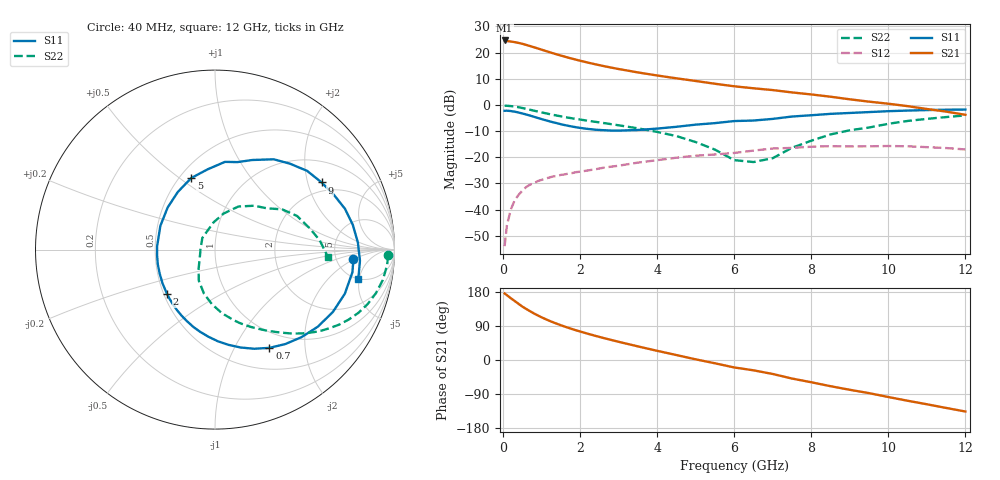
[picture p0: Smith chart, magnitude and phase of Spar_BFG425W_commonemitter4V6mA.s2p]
! Filename: 46bfg425.001
! BFG425W Field C1
! V1=8.248E-001V,V2=4.000E+000V, I1=6.283E-005A, I2=6.010E-003A
# GHz  S  MA  R 50
!  S11  S21  S12  S22
!Freq(GHz)  Mag  Ang  Mag  Ang  Mag  Ang  Mag  Ang
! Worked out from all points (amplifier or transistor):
!   44 points, 40 MHz to 12 GHz, reference 50 ohm
!   highest |S21| = 24.6 dB at 40 MHz (marker M1)
!   |S21| within 3 dB of that: start of sweep to 889.8 MHz
!   unconditionally stable (mu >= 1): 2.289 GHz to end of sweep
!   at 700 MHz: K = 0.40, MSG = 26.5 dB, |S12| = -30.5 dB
!   at 2.4 GHz: K = 1.03, MAG = 19.0 dB, |S12| = -24.6 dB
!   at 12 GHz: K = 1.47, MAG = 2.6 dB, |S12| = -17.0 dB
!   S11 on the Smith chart (normalised r, x): 40 MHz: 7.30, -1.91; 700 MHz: 0.77, -1.40; 2 GHz: 0.52, -0.30; 5 GHz: 0.57, +0.55; 9 GHz: 1.66, +2.45; 12 GHz: 5.00, -4.85
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0.04  0.773 -3.9  17.05 175.5  0.002 49.5  0.965 -1.9
0.2  0.764 -18.8  16.29 163.2  0.01 72.7  0.95 -10.3
0.4  0.716 -36.9  15.32 148.3  0.019 66.1  0.903 -19.6
0.5  0.686 -45.3  14.73 141.1  0.023 62.6  0.873 -23.8
0.7  0.626 -61.0  13.33 128.7  0.03 56.0  0.809 -31.1
0.8  0.594 -68.4  12.66 123.0  0.032 53.4  0.777 -34.2
1  0.536 -81.9  11.37 112.6  0.037 49.0  0.72 -39.6
1.3  0.466 -100.1  9.697 99.4  0.043 43.9  0.646 -46.4
1.6  0.412 -117.0  8.365 88.1  0.047 40.4  0.587 -51.9
2  0.364 -137.2  6.99 75.2  0.053 37.0  0.525 -58.6
2.2  0.348 -147.1  6.442 69.3  0.056 35.5  0.499 -61.9
3  0.323 176.6  4.854 48.0  0.069 29.6  0.408 -75.0
3.5  0.332 156.4  4.18 35.9  0.079 25.1  0.357 -83.7
4.5  0.382 122.9  3.225 13.1  0.098 14.1  0.254 -103.9
5  0.42 108.4  2.866 1.7  0.107 6.8  0.195 -117.6
6  0.492 83.5  2.27 -19.7  0.121 -7.4  0.088 -161.0
6.5  0.503 75.7  2.08 -27.2  0.134 -8.9  0.081 179.7
7.5  0.6 57.0  1.733 -48.9  0.151 -28.0  0.152 93.1
8.5  0.675 40.6  1.435 -69.2  0.163 -45.1  0.273 61.5
9  0.702 32.2  1.28 -78.6  0.161 -53.4  0.328 48.2
10.5  0.78 10.2  0.948 -107.6  0.162 -80.7  0.494 22.3
12  0.815 -11.5  0.647 -135.9  0.141 -111.7  0.63 -3.7
